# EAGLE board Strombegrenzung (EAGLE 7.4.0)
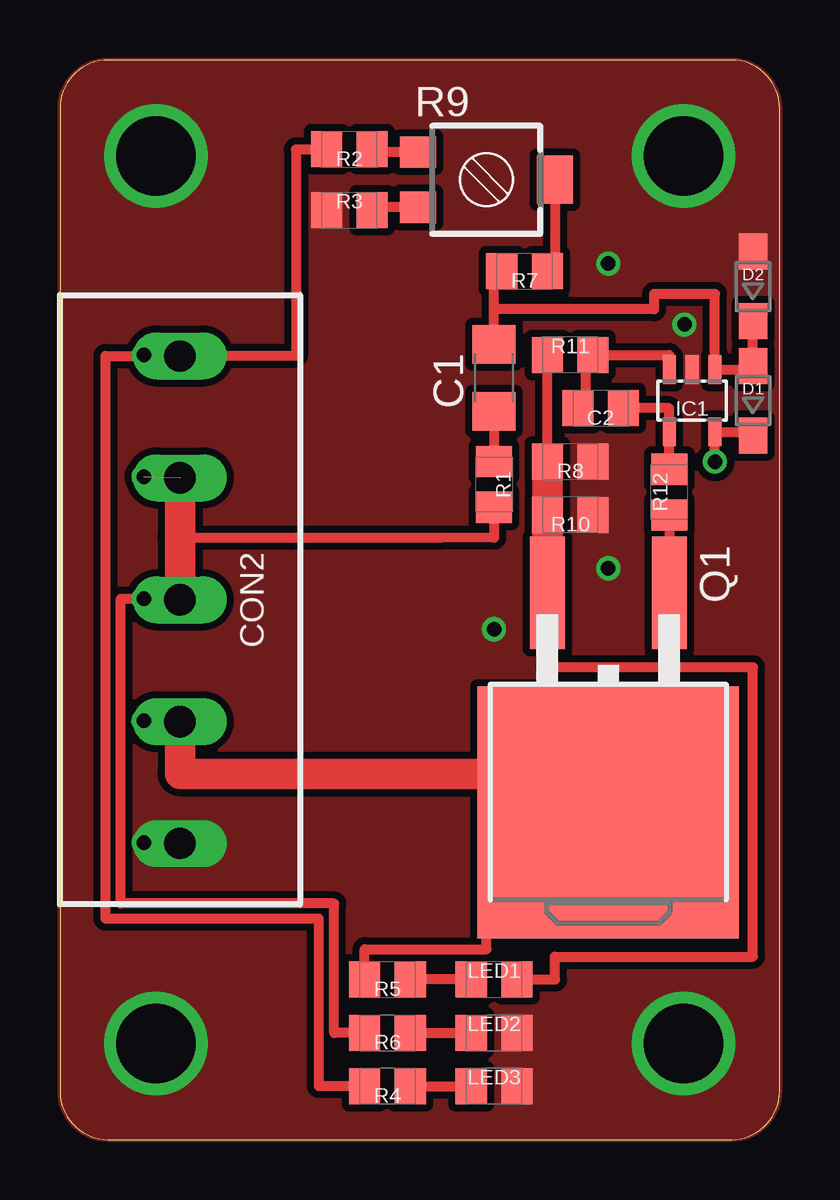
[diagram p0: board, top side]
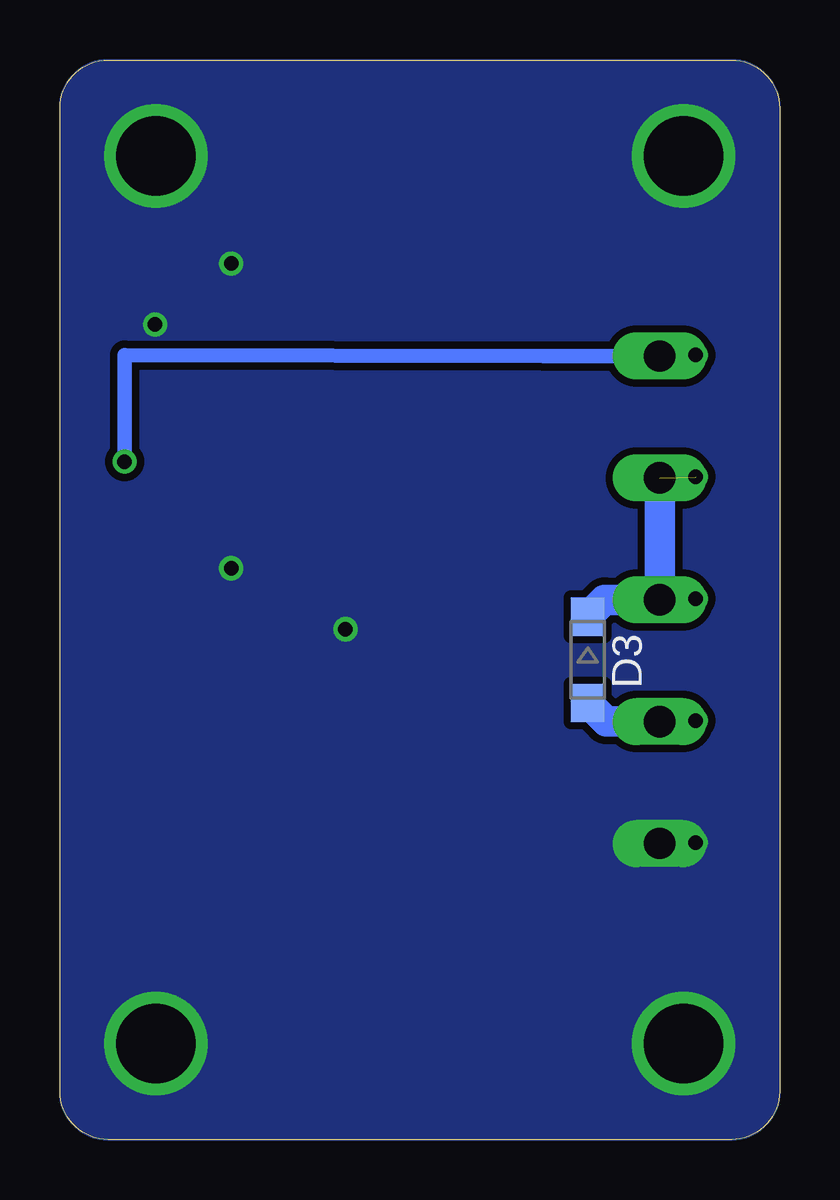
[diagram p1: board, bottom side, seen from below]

Size 30 x 45 mm. Coordinates in mm from the lower left corner, seen from the top.
Outline: 2,0 28,0 arc90 30,2 30,43 arc90 28,45 2,45 arc90 0,43 0,2 arc90 2,0
Copper layers (1*16): Top 0.035mm / dielectric 1.5mm / Bottom 0.035mm
Design rules "default *": minimum track width 10mil, minimum drill 0.6mm, track to track 8mil, track to pad 8mil, pad to pad 8mil, via to via 8mil, smd to smd 8mil, copper to edge 0mil, drill to drill 8mil, minimum pad ring 10mil, minimum via ring 8mil, stop-mask expansion 4mil, vias tented up to drill 0mil, thermal gap 10mil

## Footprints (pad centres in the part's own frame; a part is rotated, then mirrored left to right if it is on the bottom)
C1206 = smd 1.6 x 1.8: 1 -1.4,0; 2 1.4,0
C0805 = smd 1.3 x 1.5: 1 -0.95,0; 2 0.95,0
200MIL_5X = drill 1.3 long: 1 -10.16,0; 2 -5.08,0; 3 0,0; 4 5.08,0; 5 10.16,0
SOD323 = smd 1.5 x 1.2: A 1.45,0; C -1.45,0
MINI2-F3-B = smd 1.6 x 1.4: A 1.8,0; C -1.8,0
SOT-23-5 = smd 0.55 x 1.2: 1 -0.95,-1.3; 2 0,-1.3; 3 0.95,-1.3; 4 0.95,1.3; 5 -0.95,1.3
LED0805 = smd 1.3 x 1.5: A -0.95,0; C 0.95,0
TO263-3 = smd 1.45 x 4.7: 1 -2.54,-5.65; 3 2.54,-5.65 | smd 10.9 x 10.5: TAB 0,3.5
R0805 = smd 1.3 x 1.5: 1 -0.95,0; 2 0.95,0
RTRIM3314G = smd 1.3 x 1.5: CCW 1.15,-2.85; CW -1.15,-2.85 | smd 2 x 1.5: WIPER 0,2.85
HOLE_3.3MM = drill 3.3: P$1 0,0

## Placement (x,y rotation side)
C1  10u  [C1206]  18.1,31.75 90 top
C2  10n  [C0805]  22.54,30.48 180 top
CON2  CON_5X13L  [200MIL_5X]  5,22.5 270 top
D1  SCHOTTKYSOD323  [SOD323]  28.89,30.8 90 top
D2  SCHOTTKYSOD323  [SOD323]  28.89,35.56 90 top
D3  SCHOTTKYMINI2  [MINI2-F3-B]  8,20 270 bottom
IC1  LM321  [SOT-23-5]  26.35,30.8 180 top
LED1  [LED0805]  18.1,6.67 0 top
LED2  [LED0805]  18.1,4.45 0 top
LED3  [LED0805]  18.1,2.22 0 top
Q1  IPB136N08N3  [TO263-3]  22.86,17.14 180 top
R1  330  [R0805]  18.1,27.3 270 top
R2  22k  [R0805]  12.06,41.27 180 top
R3  330  [R0805]  12.06,38.73 0 top
R4  2k  [R0805]  13.65,2.22 180 top
R5  2k  [R0805]  13.65,6.67 180 top
R6  5k1  [R0805]  13.65,4.45 180 top
R7  100k  [R0805]  19.37,36.2 180 top
R8  10  [R0805]  21.27,28.26 180 top
R9  1k  [RTRIM3314G]  17.78,40.01 270 top
R10  10  [R0805]  21.27,26.04 180 top
R11  5k1  [R0805]  21.27,32.7 0 top
R12  330  [R0805]  25.4,26.99 90 top
U$1  HOLE_3.3MM  [HOLE_3.3MM]  4,41 0 top
U$2  HOLE_3.3MM  [HOLE_3.3MM]  4,4 0 top
U$3  HOLE_3.3MM  [HOLE_3.3MM]  26,41 0 top
U$4  HOLE_3.3MM  [HOLE_3.3MM]  26,4 0 top

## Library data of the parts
C1 C2 = 00Capacitor
CON2 = 00Connector
D1-D3 = 00Diode
IC1 = 00OpAmp
LED1-LED3 = 00Display
Q1 = 00Mosfet
R1-R12 = 00Resistor
U$1-U$4 = 00Drill

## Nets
+12V: CON2.1 D1.C IC1.5 R2.2 R4.2
GND: CON2.5 D2.A IC1.2 LED2.C LED3.C R3.1 R8.1 R10.1 U$1.P$1 U$2.P$1 U$3.P$1 U$4.P$1
N$1: C1.1 R1.1
N$2: R7.1 R9.WIPER
N$3: C1.2 D1.A D2.C IC1.1 R7.2
N$4: Q1.1 R12.1
N$5: LED1.A R5.1
N$6: LED3.A R4.1
N$7: C2.2 IC1.3 R11.2
N$8: R2.1 R9.CW
N$9: R3.2 R9.CCW
N$10: C2.1 IC1.4 R12.2
N$20: LED1.C Q1.3 R8.2 R10.2 R11.1
R6: LED2.A R6.1
RELAIS+: CON2.2 CON2.3 D3.C R1.2 R6.2
RELAIS-: CON2.4 D3.A Q1.TAB R5.2

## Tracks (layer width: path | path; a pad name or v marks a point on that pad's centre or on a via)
+12V  (via drill 0.6)
  Top 0.406: 28.89,29.5 IC1.5 27.3,28.57 v27.3,28.26 | R2.2 9.84,41.27 9.84,32.66 CON2.1 | R4.2 10.79,2.22 10.79,9.21 1.91,9.21 1.91,32.66 CON2.1 | v3.49,32.7 3.17,32.66 CON2.1
  Top 0.61: 28.89,29.5 D1.C
  Bottom 0.61: CON2.1 9.84,32.66 27.3,32.7 v27.3,28.26
GND  (via drill 0.6)
  other vias: 22.86,23.81 3.49,12.38 18.1,21.27 22.86,36.51 26.04,33.97
  pour Top (isolate 0.3, no thermals): 0,2 0,43 arc-90 2,45 28,45 arc-90 30,43 30,2 arc-90 28,0 2,0 arc-90
  pour Bottom (isolate 0.305, no thermals): 0,40 0,43 arc-90 2,45 15,45 28,45 arc-90 30,43 30,25 30,2 arc-90 28,0 15,0 2,0 arc-90 0,2
N$1
  Top 0.406: C1.1 R1.1
N$2
  Top 0.406: R9.WIPER 20.64,36.2 R7.1
N$3
  Top 0.406: 28.89,32.1 IC1.1 27.3,35.24 24.77,35.24 24.77,34.61 18.1,34.61 | D1.A D2.C | C1.2 18.1,34.61 | 18.1,34.61 18.1,36.2 R7.2
  Top 0.61: 28.89,32.1 D1.A
N$4
  Top 0.406: R12.1 Q1.1
N$5
  Top 0.406: LED1.A R5.1
N$6
  Top 0.406: R4.1 LED3.A
N$7
  Top 0.406: C2.2 21.91,30.48 21.91,32.7 R11.2 25.4,32.7 IC1.3
N$8
  Top 0.406: R9.CW 13.02,41.16 R2.1
N$9
  Top 0.406: R9.CCW 13.02,38.85 R3.2
N$10
  Top 0.406: R12.2 IC1.4 25.4,30.48 C2.1
N$20
  Top 0.406: LED1.C 20.64,6.67 20.64,7.62 28.89,7.62 28.89,19.68 20.32,19.68 Q1.3 | R8.2 R11.1
  Top 1.27: R8.2 R10.2 20.32,26.35 Q1.3
R6
  Top 0.406: R6.1 LED2.A
RELAIS+  (via drill 0.6)  (1 unrouted)
  Top 0.406: R6.2 11.43,4.45 11.43,9.84 2.54,9.84 2.54,22.54 v3.49,22.54 5,22.54 | R1.2 18.1,25.09 15.88,25.08 5,25.08
  Top 1.27: CON2.2 5,25.08 5,22.54 CON2.3
  Bottom 1.27: CON2.2 5,22.54 5.08,22.54 | D3.C 7.3,22.5 CON2.3
  other vias: 3.49,27.62
RELAIS-  (via drill 0.6)
  Top 0.406: R5.2 12.7,7.94 17.78,7.94 17.78,9.53 18.41,14.6 18.73,14.6 Q1.TAB | v3.49,17.46 3.17,17.42 CON2.4
  Top 0.61: 18.73,15.24 18.73,14.6
  Top 1.27: CON2.4 5,15.24 18.73,15.24
  Bottom 1.27: D3.A 7.22,17.42 CON2.4

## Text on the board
tText: 12V | IN | R+ | R- | GND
